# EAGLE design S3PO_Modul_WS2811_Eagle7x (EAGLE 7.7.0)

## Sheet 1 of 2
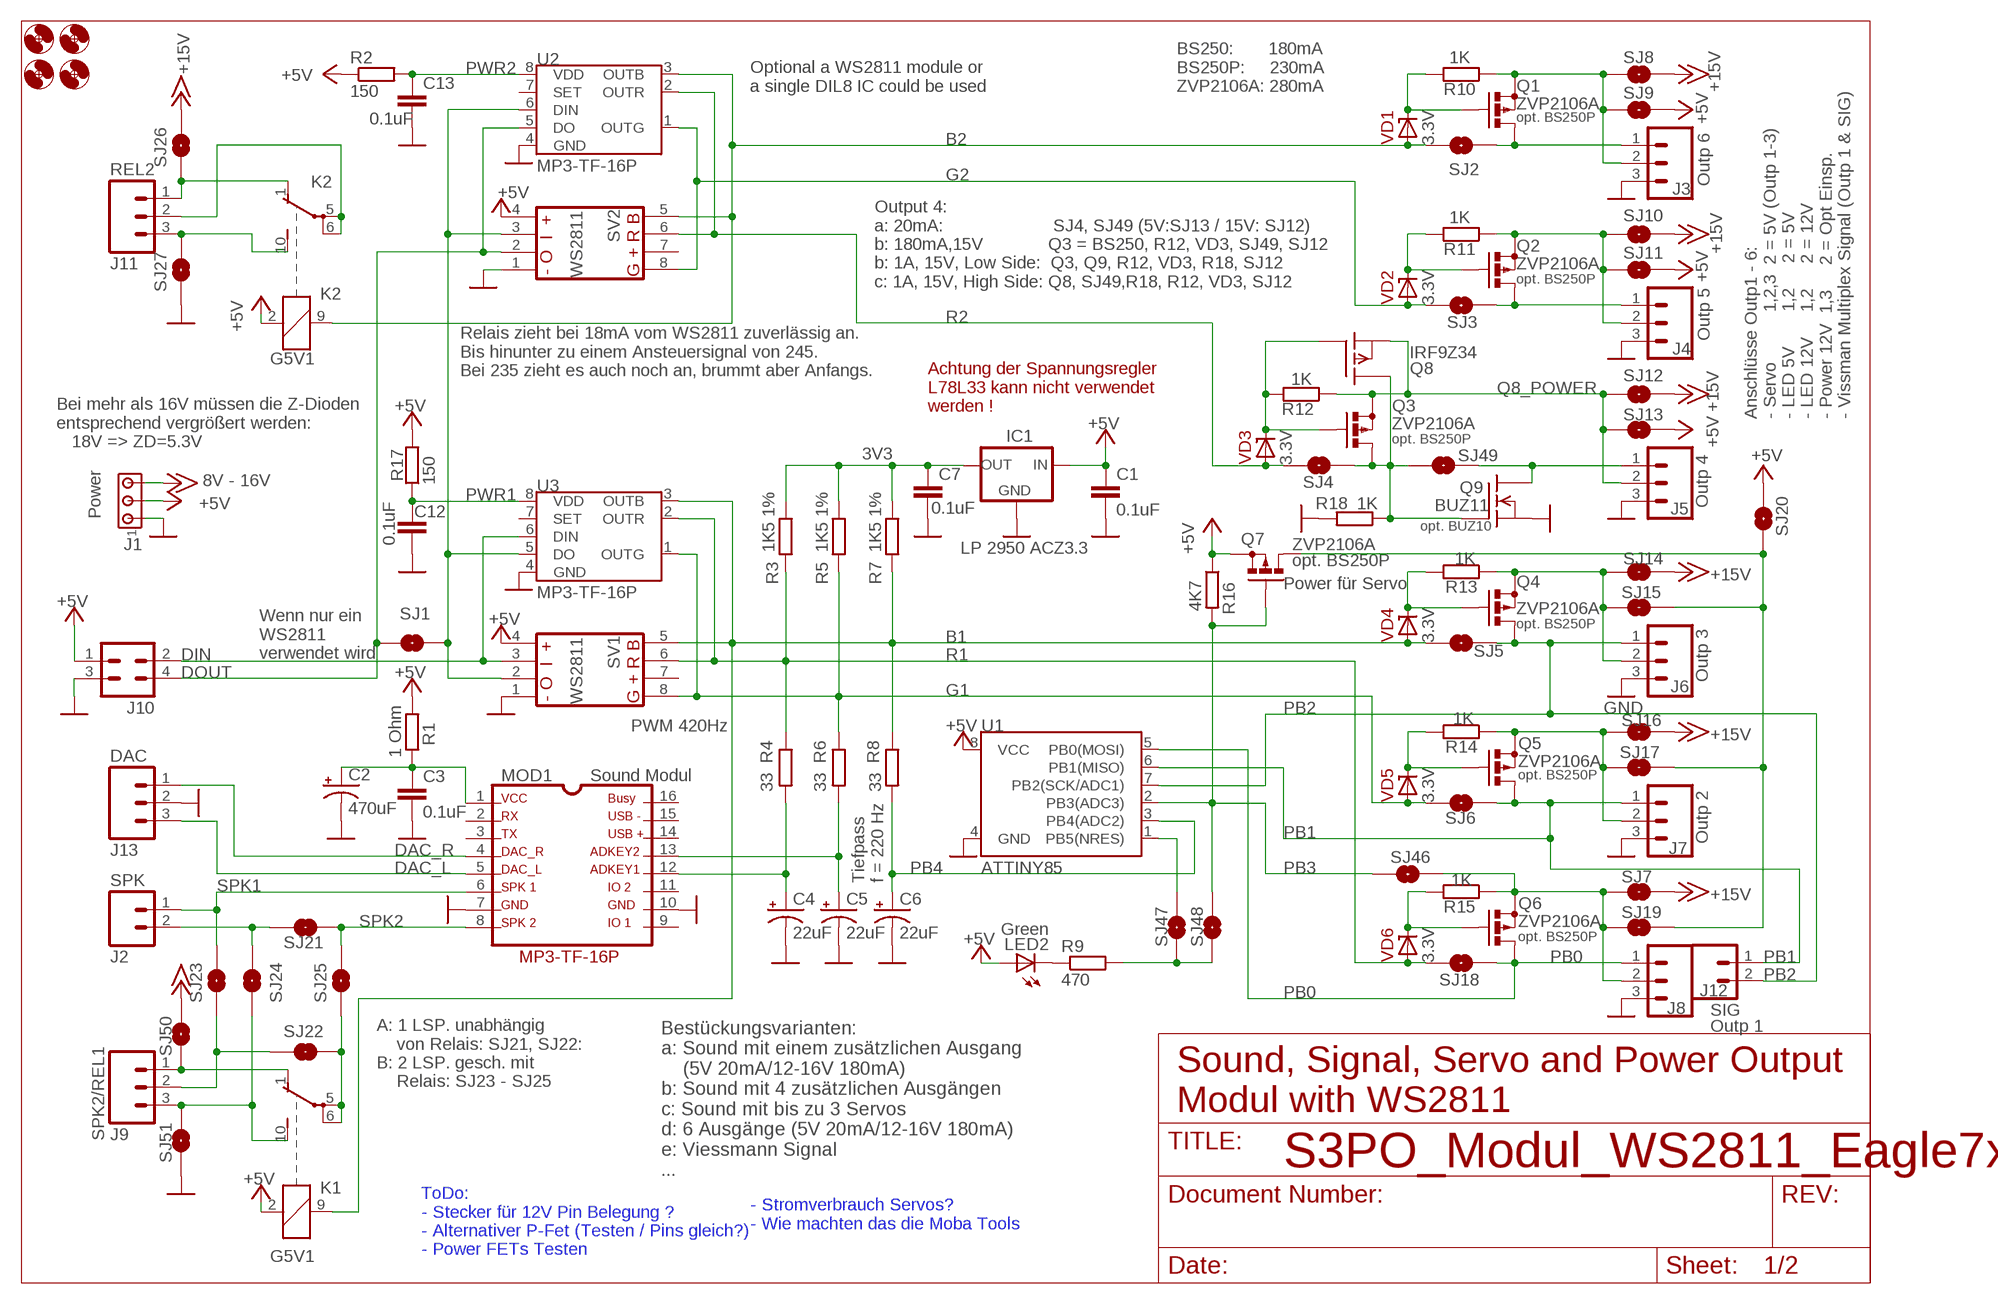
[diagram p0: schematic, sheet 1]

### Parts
C1  0.1uF  0.1UF-50V-20%(PTH)KIT-EZ  [CAP-PTH-SMALL-KIT]
C2  470uF  SPARKFUN-CAPACITORS_100UF-25V-20%(PTH)  [SPARKFUN-CAPACITORS_CPOL-RADIAL-100UF-25V]
C3  0.1uF  0.1UF-50V-20%(PTH)KIT-EZ  [CAP-PTH-SMALL-KIT]
C4  22uF  CAPACITORS_22UF  [CAPACITOR_CPOL-RADIAL-22UF]
C5  22uF  CAPACITORS_22UF  [CAPACITOR_CPOL-RADIAL-22UF]
C6  22uF  CAPACITORS_22UF  [CAPACITOR_CPOL-RADIAL-22UF]
C7  0.1uF  0.1UF-50V-20%(PTH)KIT-EZ  [CAP-PTH-SMALL-KIT]
C12  0.1uF  0.1UF-50V-20%(PTH)KIT-EZ  [CAP-PTH-SMALL-KIT]
C13  0.1uF  0.1UF-50V-20%(PTH)KIT-EZ  [CAP-PTH-SMALL-KIT]
H1  MOUNT-HOLE3.0  [3,0]
H2  MOUNT-HOLE3.0  [3,0]
H3  MOUNT-HOLE3.0  [3,0]
H4  MOUNT-HOLE3.0  [3,0]
IC1  LP 2950 ACZ3.3  78LXX  [78LXX]
J1  Power  MTA03-100  [10X03MTA]
J2  SPK  M02PTH  [1X02]
J3  Outp 6  M03PTH  [1X03]
J4  Outp 5  M03PTH  [1X03]
J5  Outp 4  M03PTH  [1X03]
J6  Outp 3  M03PTH  [1X03]
J7  Outp 2  M03PTH  [1X03]
J8  Outp 1  M03PTH  [1X03]
J9  SPK2/REL1  M03PTH  [1X03]
J10  INP  CON-HARTING-ML_ML4  [CON-HARTING-ML_ML4]
J11  REL2  M03PTH  [1X03]
J12  SIG  M02PTH  [1X02]
J13  DAC  M03PTH  [1X03]
K1  G5V1  [G5V1]
K2  G5V1  [G5V1]
LED2  Green  LED_LED3MM  [LED_LED3MM]
MOD1  Sound Modul  MP3-TF-16P_MP3-TF-16P  [MP3-TF-16P_MP3-TF-16P]
Q1  ZVP2106A  BS250  [SOT54E]
Q2  ZVP2106A  BS250  [SOT54E]
Q3  ZVP2106A  BS250  [SOT54E]
Q4  ZVP2106A  BS250  [SOT54E]
Q5  ZVP2106A  BS250  [SOT54E]
Q6  ZVP2106A  BS250  [SOT54E]
Q7  ZVP2106A  BS250  [SOT54E]
Q8  IRF9Z34  P-FET_IRF9Z34V  [TO220V]
Q9  BUZ11  N-FET_BUZ11V  [TO220V]
R1  1 Ohm  RCL_R-EU_0207/2V  [RCL_0207/2V]
R2  150  RCL_R-EU_0207/2V  [RCL_0207/2V]
R3  1K5 1%  RCL_R-EU_0204/5  [RCL_0204/5]
R4  33  RCL_R-EU_0204/5  [RCL_0204/5]
R5  1K5 1%  RCL_R-EU_0204/5  [RCL_0204/5]
R6  33  RCL_R-EU_0204/5  [RCL_0204/5]
R7  1K5 1%  RCL_R-EU_0204/5  [RCL_0204/5]
R8  33  RCL_R-EU_0204/5  [RCL_0204/5]
R9  470  RCL_R-EU_0207/2V  [RCL_0207/2V]
R10  1K  RCL_R-EU_0207/2V  [RCL_0207/2V]
R11  1K  RCL_R-EU_0207/2V  [RCL_0207/2V]
R12  1K  RCL_R-EU_0207/2V  [RCL_0207/2V]
R13  1K  RCL_R-EU_0207/2V  [RCL_0207/2V]
R14  1K  RCL_R-EU_0207/2V  [RCL_0207/2V]
R15  1K  RCL_R-EU_0207/2V  [RCL_0207/2V]
R16  4K7  RCL_R-EU_0207/2V  [RCL_0207/2V]
R17  150  RCL_R-EU_0207/2V  [RCL_0207/2V]
R18  1K  RCL_R-EU_0204/7  [RCL_0204/7]
SJ1  SOLDERJUMPERNO  [SJ_2S-NO]
SJ2  SOLDERJUMPERNO  [SJ_2S-NO]
SJ3  SOLDERJUMPERNO  [SJ_2S-NO]
SJ4  SOLDERJUMPERNO  [SJ_2S-NO]
SJ5  SOLDERJUMPERNO  [SJ_2S-NO]
SJ6  SOLDERJUMPERNO  [SJ_2S-NO]
SJ7  SOLDERJUMPERNO  [SJ_2S-NO]
SJ8  SOLDERJUMPERNO  [SJ_2S-NO]
SJ9  SOLDERJUMPERNO  [SJ_2S-NO]
SJ10  SOLDERJUMPERNO  [SJ_2S-NO]
SJ11  SOLDERJUMPERNO  [SJ_2S-NO]
SJ12  SOLDERJUMPERNO  [SJ_2S-NO]
SJ13  SOLDERJUMPERNO  [SJ_2S-NO]
SJ14  SOLDERJUMPERNO  [SJ_2S-NO]
SJ15  SOLDERJUMPERNO  [SJ_2S-NO]
SJ16  SOLDERJUMPERNO  [SJ_2S-NO]
SJ17  SOLDERJUMPERNO  [SJ_2S-NO]
SJ18  SOLDERJUMPERNO  [SJ_2S-NO]
SJ19  SOLDERJUMPERNO  [SJ_2S-NO]
SJ20  Servo Const 5V  SOLDERJUMPERNO  [SJ_2S-NO]
SJ21  SOLDERJUMPERNO  [SJ_2S-NO]
SJ22  SOLDERJUMPERNO  [SJ_2S-NO]
SJ23  SOLDERJUMPERNO  [SJ_2S-NO]
SJ24  SOLDERJUMPERNO  [SJ_2S-NO]
SJ25  SOLDERJUMPERNO  [SJ_2S-NO]
SJ26  SOLDERJUMPERNO  [SJ_2S-NO]
SJ27  SOLDERJUMPERNO  [SJ_2S-NO]
SJ46  Servo Const 5V  SOLDERJUMPERNO  [SJ_2S-NO]
SJ47  SOLDERJUMPERNO  [SJ_2S-NO]
SJ48  SOLDERJUMPERNO  [SJ_2S-NO]
SJ49  SOLDERJUMPERNO  [SJ_2S-NO]
SJ50  SOLDERJUMPERNO  [SJ_2S-NO]
SJ51  SOLDERJUMPERNO  [SJ_2S-NO]
SV1  S3PO_MODUL_WS2811_SOUND_MP3-TF-16P_WS2811_AND_ATTINY_PUSHBUTTONACTION_4017_2_WS28115V  [S3PO_MODUL_WS2811_SOUND_MP3-TF-16P_WS2811_AND_ATTINY_PUSHBUTTONACTION_4017_2_WS2811_WS2811_5V]
SV2  S3PO_MODUL_WS2811_SOUND_MP3-TF-16P_WS2811_AND_ATTINY_PUSHBUTTONACTION_4017_2_WS28115V  [S3PO_MODUL_WS2811_SOUND_MP3-TF-16P_WS2811_AND_ATTINY_PUSHBUTTONACTION_4017_2_WS2811_WS2811_5V]
U1  ATTINY85  ATTINY45TINY85-20-DIP  [DIP08]
U2  MP3-TF-16P  S3PO_MODUL_WS2811_SOUND_MP3-TF-16P_WS2811_AND_ATTINY_WS2811-ICTINY45-20-DIP  [S3PO_MODUL_WS2811_SOUND_MP3-TF-16P_WS2811_AND_ATTINY_WS2811_DIP08]
U3  MP3-TF-16P  S3PO_MODUL_WS2811_SOUND_MP3-TF-16P_WS2811_AND_ATTINY_WS2811-ICTINY45-20-DIP  [S3PO_MODUL_WS2811_SOUND_MP3-TF-16P_WS2811_AND_ATTINY_WS2811_DIP08]
VD1  3.3V  DIODES-ZENER_10V(1N4740)  [DIODES-ZENER_207/2V]
VD2  3.3V  DIODES-ZENER_10V(1N4740)  [DIODES-ZENER_207/2V]
VD3  3.3V  DIODES-ZENER_10V(1N4740)  [DIODES-ZENER_207/2V]
VD4  3.3V  DIODES-ZENER_10V(1N4740)  [DIODES-ZENER_207/2V]
VD5  3.3V  DIODES-ZENER_10V(1N4740)  [DIODES-ZENER_207/2V]
VD6  3.3V  DIODES-ZENER_10V(1N4740)  [DIODES-ZENER_207/2V]

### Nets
3V3: C7.1 IC1.OUT R3.1 R5.1 R7.1
+5V: C1.1 IC1.IN J1.2 J10.1 K1.2 K2.2 LED2.A Q7.S R1.1 R2.1 R16.1 R17.2 SJ9.2 SJ11.2 SJ13.2 SJ20.2 SV1.4(GND) SV2.4(GND) U1.8(VCC)
+15V: J1.3 SJ7.2 SJ8.2 SJ10.2 SJ12.2 SJ14.2 SJ16.2 SJ26.1 SJ50.1
B1: K1.9 R7.2 R8.1 SJ5.2 SV1.5(OUTG) U3.3(OUTB) VD4.A
B2: K2.9 SJ2.2 SV2.5(OUTG) U2.3(OUTB) VD1.A
DAC_L: J13.3 MOD1.5
DAC_R: J13.1 MOD1.4
DIN: J10.2 SV1.3(DO) U3.6(DIN)
DOUT: J10.4 SJ1.2 SV2.2(DIN) U2.5(DO)
G1: R5.2 R6.1 SJ6.2 SV1.8(OUTB) U3.1(OUTG) VD5.A
G2: SJ3.2 SV2.8(OUTB) U2.1(OUTG) VD2.A
GND: C1.2 C2.2(-) C3.2 C4.2(-) C5.2(-) C6.2(-) C7.2 C12.2 C13.2 IC1.GND J1.1 J3.3 J4.3 J5.3 J6.3 J7.3 J8.3 J10.3 J13.2 MOD1.7 MOD1.10 Q9.3(S) R18.2 SJ27.2 SJ51.2 SV1.1(VDD) SV2.1(VDD) U1.4(GND) U2.4(GND) U3.4(GND)
N$4: SJ1.1 SV1.2(DIN) SV2.3(DO) U2.6(DIN) U3.5(DO)
N$6: LED2.K(C) R9.1
N$7: C4.1(+) MOD1.12 R4.2
N$8: C5.1(+) MOD1.13 R6.2
N$9: C2.1(+) C3.1 MOD1.1 R1.2
N$10: Q4.G R13.2 VD4.C
N$14: J5.1 Q9.2(D) SJ49.2
N$17: Q6.G R15.2 VD6.C
N$18: Q3.D Q8.2(D) Q9.1(G) R18.1 SJ4.1 SJ49.1
N$19: Q3.G Q8.1(G) R12.2 VD3.C
N$21: J2.2 SJ21.2 SJ24.1
N$22: J4.1 Q2.D SJ3.1
N$23: Q2.G R11.2 VD2.C
N$24: J7.2 Q5.S R14.1 SJ16.1 SJ17.1
N$25: J8.2 Q6.S R15.1 SJ7.1 SJ19.1 SJ46.2
N$26: J3.1 Q1.D SJ2.1
N$27: Q1.G R10.2 VD1.C
N$29: K1.5(2:P) K1.6(2:P) SJ22.1 SJ25.2
N$32: Q5.G R14.2 VD5.C
N$34: J9.3 K1.10(2:S) SJ24.2 SJ51.1
N$35: J9.1 K1.1(2:O) SJ50.2
N$36: J9.2 SJ22.2 SJ23.2
N$37: J6.2 Q4.S R13.1 SJ14.1 SJ15.1
N$41: J4.2 Q2.S R11.1 SJ10.1 SJ11.1
N$42: J3.2 Q1.S R10.1 SJ8.1 SJ9.1
N$43: J11.2 K2.5(2:P) K2.6(2:P)
N$44: Q7.D SJ15.2 SJ17.2 SJ19.2 SJ20.1
N$45: J11.3 K2.10(2:S) SJ27.1
N$46: J11.1 K2.1(2:O) SJ26.2
N$70: SJ47.2 U1.1(PB5(NRES))
N$74: R9.2 SJ47.1 SJ48.2
PB0: J8.1 Q6.D SJ18.1 U1.5(PB0(MOSI))
PB1: J7.1 J12.1 Q5.D SJ6.1 U1.6(PB1(MISO))
PB2: J6.1 J12.2 Q4.D SJ5.1 U1.7(PB2(SCK/ADC1))
PB3: Q7.G R16.2 SJ46.1 SJ48.1 U1.2(PB3(ADC3))
PB4: C6.1(+) R8.2 U1.3(PB4(ADC2))
PWR1: C12.1 R17.1 U3.8(VDD)
PWR2: C13.1 R2.2 U2.8(VDD)
Q8_POWER: J5.2 Q3.S Q8.3(S) R12.1 SJ12.1 SJ13.1
R1: R3.2 R4.1 SJ18.2 SV1.6(OUT+) U3.2(OUTR) VD6.A
R2: SJ4.2 SV2.6(OUT+) U2.2(OUTR) VD3.A
SPK1: J2.1 MOD1.6 SJ23.1
SPK2: MOD1.8 SJ21.1 SJ25.1
Unconnected: MOD1.2 MOD1.3 MOD1.9 MOD1.11 MOD1.14 MOD1.15 MOD1.16 SV1.7(OUTR) SV2.7(OUTR) U2.7(SET) U3.7(SET)

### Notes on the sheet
- Optional a WS2811 module or
  a single DIL8 IC could be used
- BS250:       180mA
  BS250P:     230mA
  ZVP2106A: 280mA
- opt. BS250P
- opt. BS250P
- Output 4:
  a: 20mA:                      SJ4, SJ49 (5V:SJ13 / 15V: SJ12) 
  b: 180mA,15V             Q3 = BS250, R12, VD3, SJ49, SJ12
  b: 1A, 15V, Low Side:  Q3, Q9, R12, VD3, R18, SJ12
  c: 1A, 15V, High Side: Q8, SJ49,R18, R12, VD3, SJ12
- Relais zieht bei 18mA vom WS2811 zuverlässig an.
  Bis hinunter zu einem Ansteuersignal von 245.
  Bei 235 zieht es auch noch an, brummt aber Anfangs.
- Achtung der Spannungsregler
  L78L33 kann nicht verwendet
  werden !
- Anschlüsse Outp1 - 6:
  - Servo          1,2,3  2 = 5V (Outp 1-3)
  - LED 5V       1,2     2 = 5V
  - LED 12V     1,2     2 = 12V
  - Power 12V  1,3     2 = Opt Einsp.
  - Vissman Multiplex Signal (Outp 1 & SIG)
- opt. BS250P
- Bei mehr als 16V müssen die Z-Dioden
  entsprechend vergrößert werden: 
     18V => ZD=5.3V
- 8V - 16V
- opt. BUZ10
- opt. BS250P
- Power für Servo
- opt. BS250P
- Wenn nur ein  
  WS2811 
  verwendet wird
- PWM 420Hz
- opt. BS250P
- Tiefpass 
  f = 220 Hz
- opt. BS250P
- A: 1 LSP. unabhängig
      von Relais: SJ21, SJ22: 
  B: 2 LSP. gesch. mit
      Relais: SJ23 - SJ25
- Sound, Signal, Servo and Power Output
  Modul with WS2811
- Bestückungsvarianten:
  a: Sound mit einem zusätzlichen Ausgang 
      (5V 20mA/12-16V 180mA)
  b: Sound mit 4 zusätzlichen Ausgängen          
  c: Sound mit bis zu 3 Servos 
  d: 6 Ausgänge (5V 20mA/12-16V 180mA)
  e: Viessmann Signal
  ...
- - Stromverbrauch Servos? 
  - Wie machten das die Moba Tools
- ToDo:
  - Stecker für 12V Pin Belegung ?
  - Alternativer P-Fet (Testen / Pins gleich?)
  - Power FETs Testen

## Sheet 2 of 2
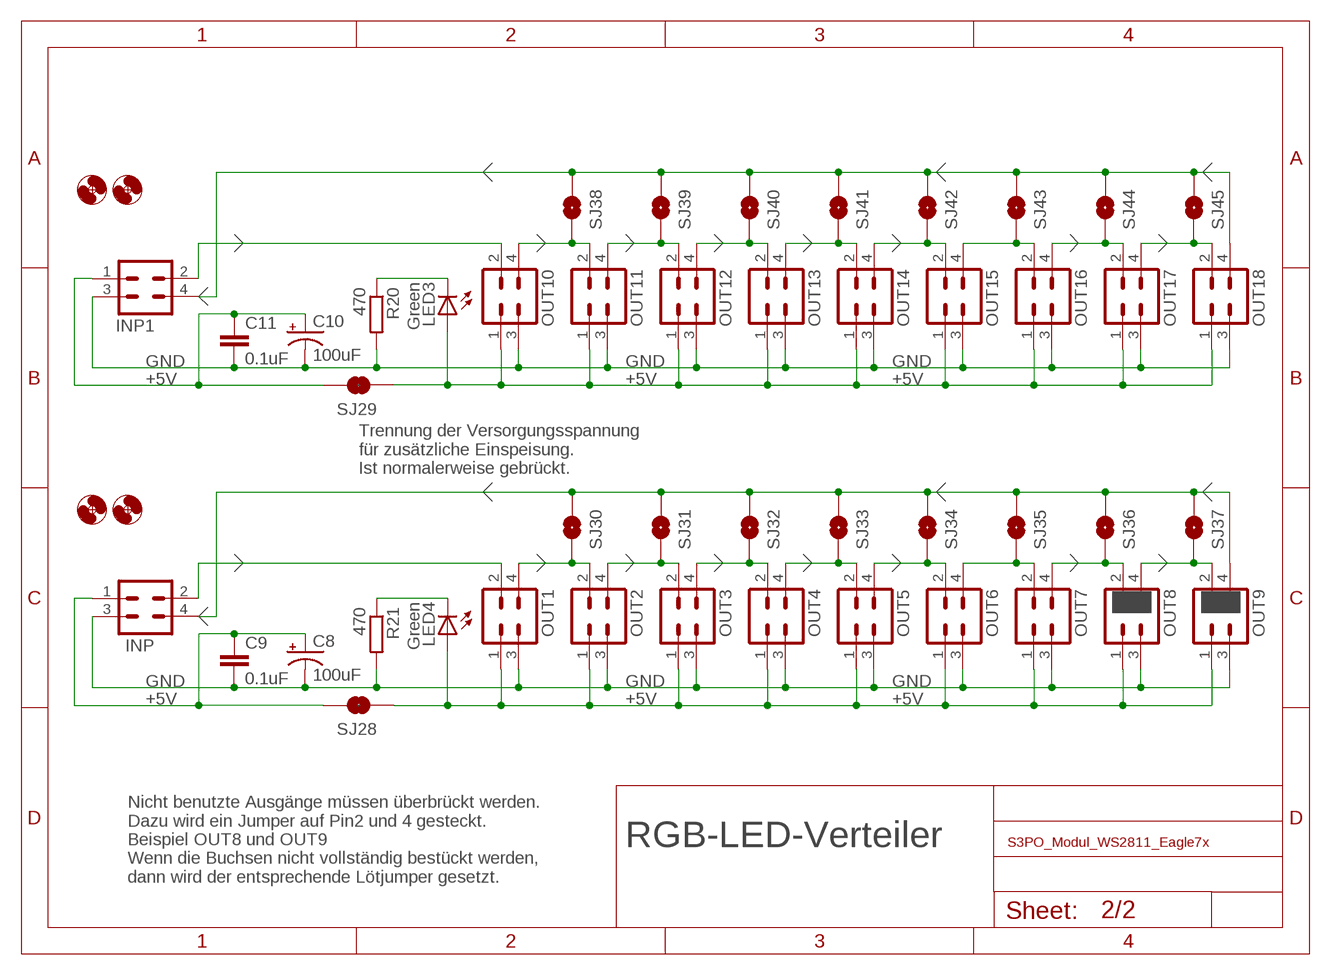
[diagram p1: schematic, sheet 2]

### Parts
C8  100uF  SPARKFUN-CAPACITORS_100UF-25V-20%(PTH)  [SPARKFUN-CAPACITORS_CPOL-RADIAL-100UF-25V]
C9  0.1uF  0.1UF-50V-20%(PTH)KIT-EZ  [CAP-PTH-SMALL-KIT]
C10  100uF  SPARKFUN-CAPACITORS_100UF-25V-20%(PTH)  [SPARKFUN-CAPACITORS_CPOL-RADIAL-100UF-25V]
C11  0.1uF  0.1UF-50V-20%(PTH)KIT-EZ  [CAP-PTH-SMALL-KIT]
H5  MOUNT-HOLE3.0  [3,0]
H6  MOUNT-HOLE3.0  [3,0]
H7  MOUNT-HOLE3.0  [3,0]
H8  MOUNT-HOLE3.0  [3,0]
INP  CON-HARTING-ML_ML4  [CON-HARTING-ML_ML4]
INP1  CON-HARTING-ML_ML4  [CON-HARTING-ML_ML4]
LED3  Green  LED_LED3MM  [LED_LED3MM]
LED4  Green  LED_LED3MM  [LED_LED3MM]
OUT1  CON-HARTING-ML_ML4  [CON-HARTING-ML_ML4]
OUT2  CON-HARTING-ML_ML4  [CON-HARTING-ML_ML4]
OUT3  CON-HARTING-ML_ML4  [CON-HARTING-ML_ML4]
OUT4  CON-HARTING-ML_ML4  [CON-HARTING-ML_ML4]
OUT5  CON-HARTING-ML_ML4  [CON-HARTING-ML_ML4]
OUT6  CON-HARTING-ML_ML4  [CON-HARTING-ML_ML4]
OUT7  CON-HARTING-ML_ML4  [CON-HARTING-ML_ML4]
OUT8  CON-HARTING-ML_ML4  [CON-HARTING-ML_ML4]
OUT9  CON-HARTING-ML_ML4  [CON-HARTING-ML_ML4]
OUT10  CON-HARTING-ML_ML4  [CON-HARTING-ML_ML4]
OUT11  CON-HARTING-ML_ML4  [CON-HARTING-ML_ML4]
OUT12  CON-HARTING-ML_ML4  [CON-HARTING-ML_ML4]
OUT13  CON-HARTING-ML_ML4  [CON-HARTING-ML_ML4]
OUT14  CON-HARTING-ML_ML4  [CON-HARTING-ML_ML4]
OUT15  CON-HARTING-ML_ML4  [CON-HARTING-ML_ML4]
OUT16  CON-HARTING-ML_ML4  [CON-HARTING-ML_ML4]
OUT17  CON-HARTING-ML_ML4  [CON-HARTING-ML_ML4]
OUT18  CON-HARTING-ML_ML4  [CON-HARTING-ML_ML4]
R20  470  RCL_R-EU_0207/2V  [RCL_0207/2V]
R21  470  RCL_R-EU_0207/2V  [RCL_0207/2V]
SJ28  SOLDERJUMPERTRACE  [SJ_2S-TRACE]
SJ29  SOLDERJUMPERTRACE  [SJ_2S-TRACE]
SJ30  SOLDERJUMPERNO  [SJ_2S-NO]
SJ31  SOLDERJUMPERNO  [SJ_2S-NO]
SJ32  SOLDERJUMPERNO  [SJ_2S-NO]
SJ33  SOLDERJUMPERNO  [SJ_2S-NO]
SJ34  SOLDERJUMPERNO  [SJ_2S-NO]
SJ35  SOLDERJUMPERNO  [SJ_2S-NO]
SJ36  SOLDERJUMPERNO  [SJ_2S-NO]
SJ37  SOLDERJUMPERNO  [SJ_2S-NO]
SJ38  SOLDERJUMPERNO  [SJ_2S-NO]
SJ39  SOLDERJUMPERNO  [SJ_2S-NO]
SJ40  SOLDERJUMPERNO  [SJ_2S-NO]
SJ41  SOLDERJUMPERNO  [SJ_2S-NO]
SJ42  SOLDERJUMPERNO  [SJ_2S-NO]
SJ43  SOLDERJUMPERNO  [SJ_2S-NO]
SJ44  SOLDERJUMPERNO  [SJ_2S-NO]
SJ45  SOLDERJUMPERNO  [SJ_2S-NO]

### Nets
5V_A: LED4.A OUT1.1 OUT2.1 OUT3.1 OUT4.1 OUT5.1 OUT6.1 OUT7.1 OUT8.1 OUT9.1 SJ28.1
5V_B: LED3.A OUT10.1 OUT11.1 OUT12.1 OUT13.1 OUT14.1 OUT15.1 OUT16.1 OUT17.1 OUT18.1 SJ29.1
GND_A: C8.2(-) C9.2 INP.3 OUT1.3 OUT2.3 OUT3.3 OUT4.3 OUT5.3 OUT6.3 OUT7.3 OUT8.3 OUT9.3 R21.2
GND_B: C10.2(-) C11.2 INP1.3 OUT10.3 OUT11.3 OUT12.3 OUT13.3 OUT14.3 OUT15.3 OUT16.3 OUT17.3 OUT18.3 R20.2
N$5: LED3.K(C) R20.1
N$11: OUT1.4 OUT2.2 SJ30.2
N$12: OUT2.4 OUT3.2 SJ31.2
N$16: LED4.K(C) R21.1
N$47: OUT3.4 OUT4.2 SJ32.2
N$48: INP.2 OUT1.2
N$49: OUT10.4 OUT11.2 SJ38.2
N$50: OUT4.4 OUT5.2 SJ33.2
N$51: OUT5.4 OUT6.2 SJ34.2
N$54: OUT11.4 OUT12.2 SJ39.2
N$55: OUT7.4 OUT8.2 SJ36.2
N$56: INP.4 OUT9.4 SJ30.1 SJ31.1 SJ32.1 SJ33.1 SJ34.1 SJ35.1 SJ36.1 SJ37.1
N$57: OUT8.4 OUT9.2 SJ37.2
N$58: OUT12.4 OUT13.2 SJ40.2
N$59: INP1.2 OUT10.2
N$60: OUT13.4 OUT14.2 SJ41.2
N$61: OUT6.4 OUT7.2 SJ35.2
N$62: OUT14.4 OUT15.2 SJ42.2
N$65: OUT16.4 OUT17.2 SJ44.2
N$66: INP1.4 OUT18.4 SJ38.1 SJ39.1 SJ40.1 SJ41.1 SJ42.1 SJ43.1 SJ44.1 SJ45.1
N$67: OUT17.4 OUT18.2 SJ45.2
N$68: OUT15.4 OUT16.2 SJ43.2
N$69: C8.1(+) C9.1 INP.1 SJ28.2
N$73: C10.1(+) C11.1 INP1.1 SJ29.2

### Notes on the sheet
- GND | GND | GND
- +5V | +5V | +5V
- Trennung der Versorgungsspannung
  für zusätzliche Einspeisung.
  Ist normalerweise gebrückt.
- GND | GND | GND
- +5V | +5V | +5V
- RGB-LED-Verteiler
- Nicht benutzte Ausgänge müssen überbrückt werden.
  Dazu wird ein Jumper auf Pin2 und 4 gesteckt.
  Beispiel OUT8 und OUT9
  Wenn die Buchsen nicht vollständig bestückt werden, 
  dann wird der entsprechende Lötjumper gesetzt.

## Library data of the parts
C1 C3 C7 C9 C11-C13 = SparkFun-Capacitors:0.1UF-50V-20%(PTH): CAP-08370; PROD_ID: CAP-08370
C2 C8 C10 = Sound_MP3-TF-16P_and_WS2811:SPARKFUN-CAPACITORS_100UF-25V-20%(PTH): CAP-08439; PROD_ID: CAP-08439
C4-C6 = Sound_MP3-TF-16P_WS2811_and_ATTiny:CAPACITORS_22UF: CAP-08439; PROD_ID: CAP-08439
H1-H8 = holes:MOUNT-HOLE: MOUNTING HOLE with drill center marker
IC1 = v-reg-3:78LXX: VOLTAGE REGULATOR
INP INP1 OUT1-OUT18 = RGB-LED-Verteiler:CON-HARTING-ML_ML4
J1 = con-amp:MTA03-100: AMP connector
J2 J12 = SparkFun-Connectors:M02: Standard 2-pin 0.1" header. Use with
J3-J9 J11 J13 = SparkFun-Connectors:M03: Header 3 Standard 3-pin 0.1" header. Use with straight break away headers (SKU : PRT-00116), right angle break away headers (PRT-00553), swiss pins (PRT-00743), machine pins (PRT-00117), and female headers (PRT-00115). Molex polarized connector foot print use with SKU : PRT-08232 with associated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
J10 = Pfostenstecker_4_u_6:CON-HARTING-ML_ML4
K1 K2 = relay:G5V1: RELAY 1 x switch, 0.5 A/125 V AC, 1 A/24 V DC , Omron; MPN: G5V-1-DC24; OC_FARNELL: 9949593; OC_NEWARK: 36M6377; SPICEPREFIX: B
LED2-LED4 = Sound_MP3-TF-16P_and_WS2811:LED_LED: LED
MOD1 = Sound_MP3-TF-16P_WS2811_and_ATTiny:MP3-TF-16P_MP3-TF-16P: MP3-TF-16P http://www.electronicoscaldas.com/datasheet/DFR0299-DFPlayer-Mini-Manual.pdf; OC_FARNELL: unknown; OC_NEWARK: unknown
Q1-Q7 = transistor-small-signal:BS250: P-CHANNEL MOS FET
Q8 = S3PO_Modul_WS2811:P-FET_IRF9Z34
Q9 = S3PO_Modul_WS2811:N-FET_BUZ11: N-Channel Enhancement MOSFET 50V; 30A; 0,040Ohm
R1-R18 R20 R21 = Sound_MP3-TF-16P_and_WS2811:RCL_R-EU_: RESISTOR, European symbol; SPICEPREFIX: R
SJ1-SJ51 = SparkFun-Retired:SOLDERJUMPER: Solder Jumper
SV1 SV2 = S3PO_Modul_WS2811:S3PO_MODUL_WS2811_SOUND_MP3-TF-16P_WS2811_AND_ATTINY_PUSHBUTTONACTION_4017_2_WS2811: Modified by Hardi
U1 = SparkFun-DigitalIC:ATTINY45: Atmel 8-pin 2/4/8kB flash uC; PROD_ID: IC-09445; VALUE: TINY85-20-DIP
U2 U3 = S3PO_Modul_WS2811:S3PO_MODUL_WS2811_SOUND_MP3-TF-16P_WS2811_AND_ATTINY_WS2811-IC: Die Pin nummern im Dokument https://cdn-shop.adafruit.com/datasheets/WS2811.pdf für R und G sind vertauscht ;-(; PROD_ID: IC-09439; VALUE: TINY45-20-DIP
VD1-VD6 = Z-Diode:DIODES-ZENER_?

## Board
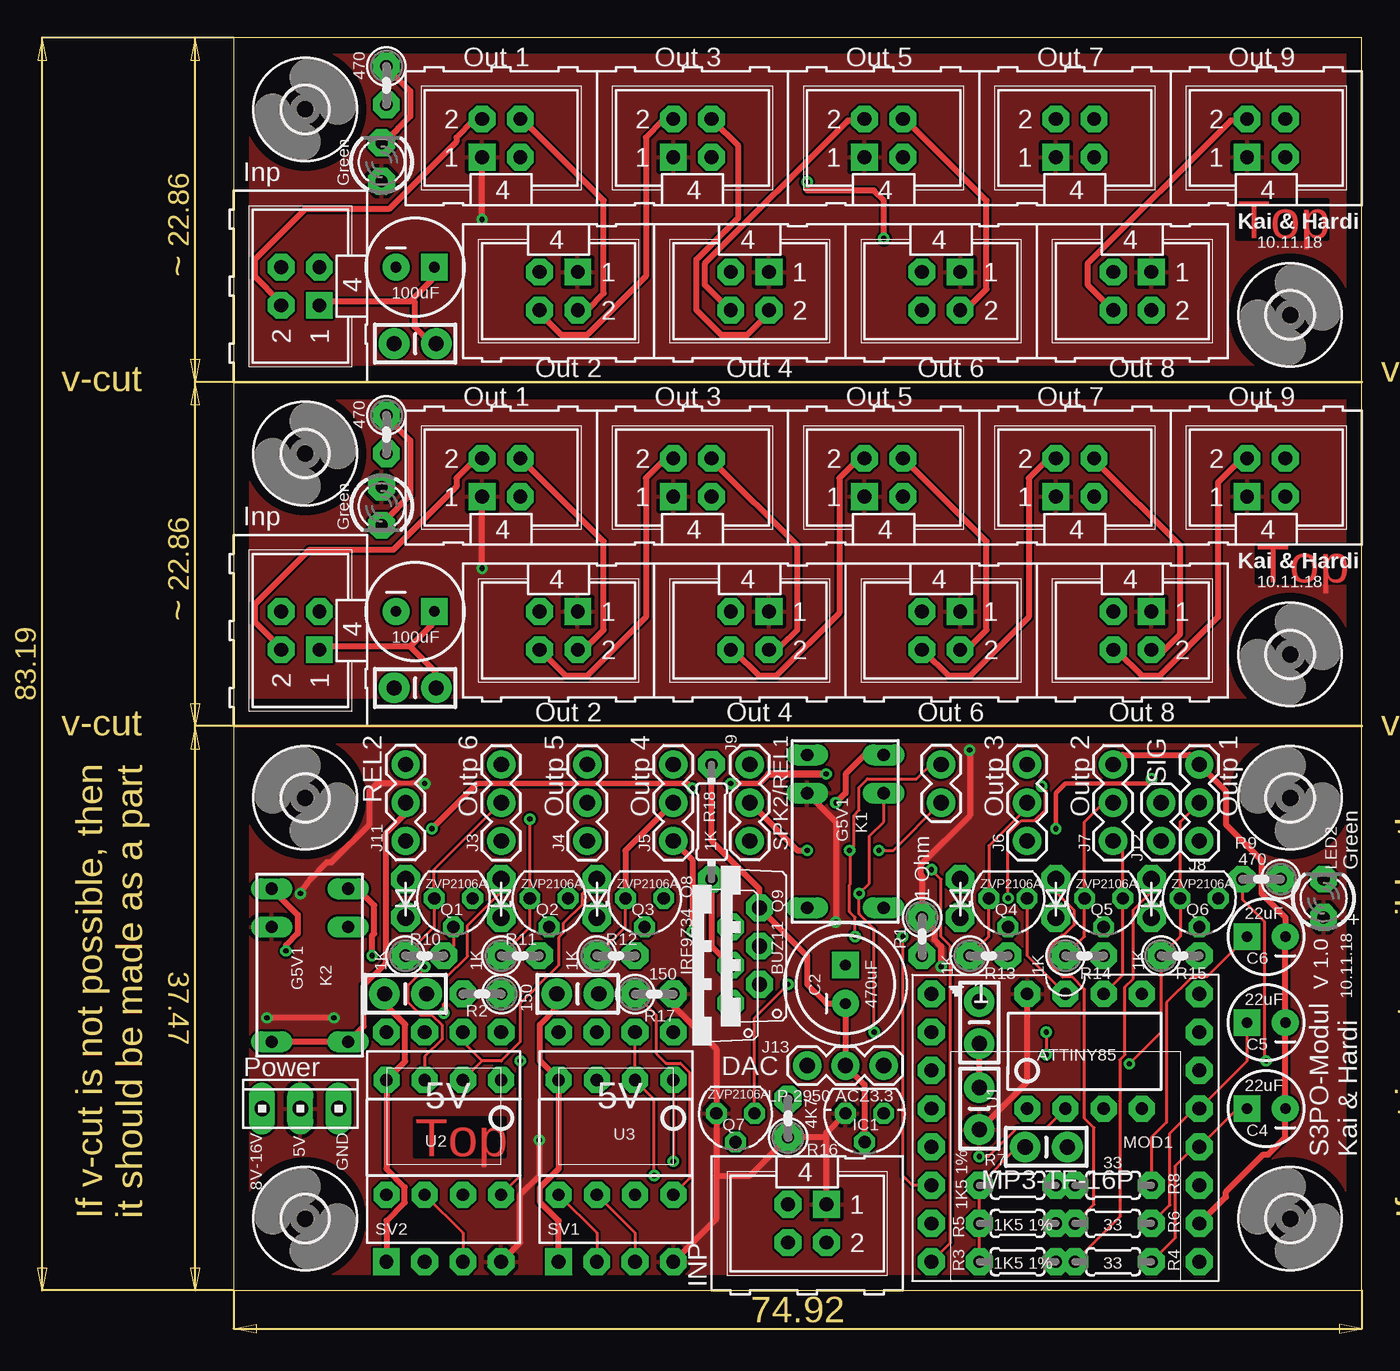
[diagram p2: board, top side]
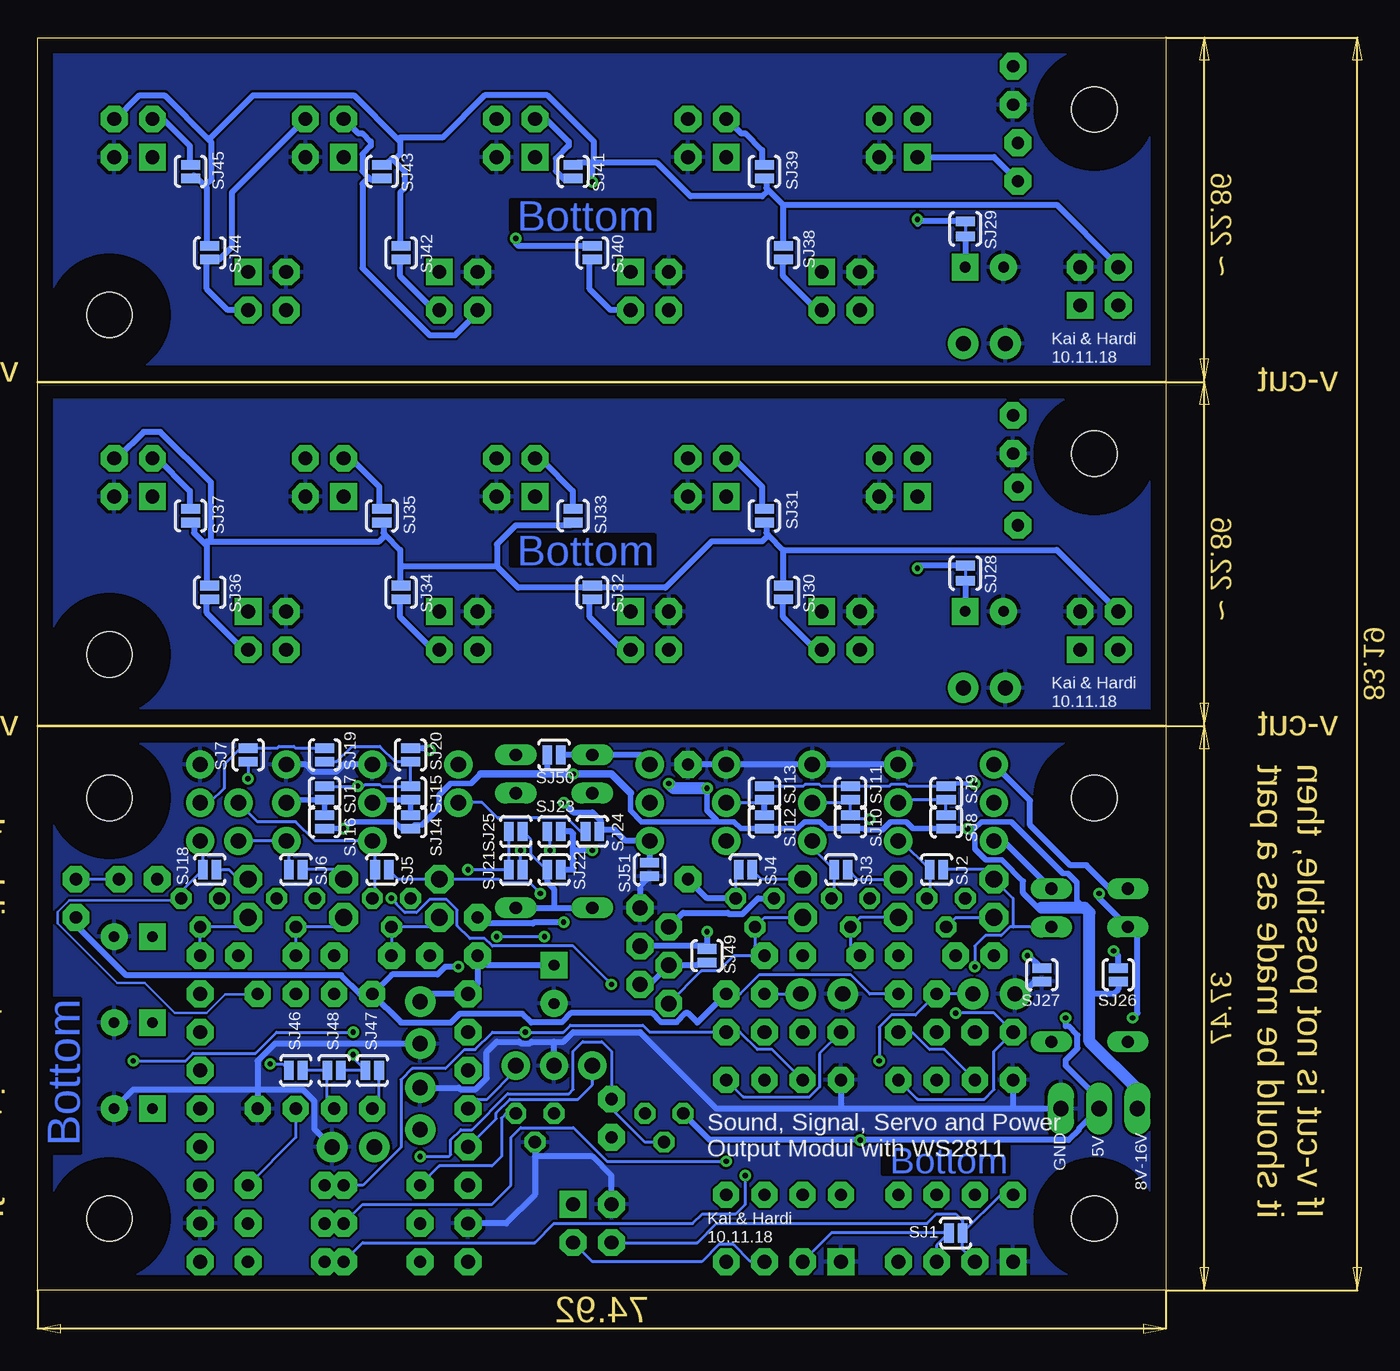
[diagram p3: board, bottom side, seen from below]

Size 87.93 x 86.03 mm. Coordinates in mm from the lower left corner, seen from the top.
Outline: 87.93,40.31 87.93,2.84 13.01,2.84 13.01,86.03 87.93,86.03 87.93,63.17
Outline: 87.93,40.31 87.93,63.17
Outline: 13,40.31 87.93,40.31
Outline: 13,63.17 87.93,63.17
Copper layers (1*16): Top 0.035mm / dielectric 1.5mm / Bottom 0.035mm
Design rules "default *": minimum track width 6mil, minimum drill 0.35mm, track to track 6mil, track to pad 6mil, pad to pad 6mil, via to via 6mil, smd to smd 6mil, copper to edge 40mil, drill to drill 6mil, minimum pad ring 10mil, minimum via ring 8mil, stop-mask expansion 4mil, vias tented up to drill 0mil, thermal gap 10mil

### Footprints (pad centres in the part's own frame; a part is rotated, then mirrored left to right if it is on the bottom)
CAP-PTH-SMALL-KIT = drill 1.016 pad 2.032: 1 -1.397,0; 2 1.397,0
SPARKFUN-CAPACITORS_CPOL-RADIAL-100UF-25V = drill 0.7 pad 1.778 square: 1 1.27,0 | drill 0.7 pad 1.778: 2 -1.27,0
CAPACITOR_CPOL-RADIAL-22UF = drill 0.7 pad 1.778 square: 1 1.27,0 | drill 0.7 pad 1.778: 2 -1.27,0
3,0 = hole 3: 0,0
78LXX = drill 0.813 octagon: GND 0,1.905; IN 1.27,0; OUT -1.27,0
CON-HARTING-ML_ML4 = drill 0.914 pad 1.778 square: 1 -2.54,-1.27 | drill 0.914 pad 1.778 octagon: 2 -2.54,1.27; 3 0,-1.27; 4 0,1.27
10X03MTA = drill 1.016 long: 1 2.54,0; 2 0,0; 3 -2.54,0
1X02 = drill 1.016 pad 1.88: 1 0,0; 2 2.54,0
1X03 = drill 1.016 pad 1.88: 1 0,0; 2 2.54,0; 3 5.08,0
G5V1 = drill 0.813 long: 1 -5.08,-2.54; 2 -2.54,-2.54; 5 5.08,-2.54; 6 5.08,2.54; 9 -2.54,2.54; 10 -5.08,2.54
LED_LED3MM = drill 0.813 pad 1.778 octagon: A -1.27,0; K 1.27,0
MP3-TF-16P_MP3-TF-16P = drill 0.914 pad 1.778 octagon: 1 -8.89,16.51; 2 -8.89,13.97; 3 -8.89,11.43; 4 -8.89,8.89; 5 -8.89,6.35; 6 -8.89,3.81; 7 -8.89,1.27; 8 -8.89,-1.27; 9 8.89,-1.27; 10 8.89,1.27; 11 8.89,3.81; 12 8.89,6.35; 13 8.89,8.89; 14 8.89,11.43; 15 8.89,13.97; 16 8.89,16.51
SOT54E = drill 0.813 octagon: D -1.27,0; G 0,1.905; S 1.27,0
TO220V = drill 1.016 pad 1.778 octagon: 1 -2.54,-2.54; 2 0,-2.54; 3 2.54,-2.54
RCL_0207/2V = drill 0.813 pad 1.778 octagon: 1 -1.27,0; 2 1.27,0
RCL_0204/5 = drill 0.813 pad 1.778 octagon: 1 -2.54,0; 2 2.54,0
RCL_0204/7 = drill 0.813 pad 1.778 octagon: 1 -3.81,0; 2 3.81,0
SJ_2S-NO = smd 0.635 x 1.27: 1 -0.45,0; 2 0.45,0
SJ_2S-TRACE = smd 0.635 x 1.27: 1 -0.508,0; 2 0.508,0
S3PO_MODUL_WS2811_SOUND_MP3-TF-16P_WS2811_AND_ATTINY_PUSHBUTTONACTION_4017_2_WS2811_WS2811_5V = drill 0.914 pad 1.778 square: 1 -5.08,-5.08 | drill 0.914 pad 1.778 octagon: 2 -2.54,-5.08; 3 0,-5.08; 4 2.54,-5.08; 5 2.54,10.16; 6 0,10.16; 7 -2.54,10.16; 8 -5.08,10.16
DIP08 = drill 0.813 pad 1.727 octagon: 1 -3.81,-3.81; 2 -1.27,-3.81; 3 1.27,-3.81; 4 3.81,-3.81; 5 3.81,3.81; 6 1.27,3.81; 7 -1.27,3.81; 8 -3.81,3.81
S3PO_MODUL_WS2811_SOUND_MP3-TF-16P_WS2811_AND_ATTINY_WS2811_DIP08 = drill 0.813 pad 1.727 octagon: 1 -3.81,-3.81; 2 -1.27,-3.81; 3 1.27,-3.81; 4 3.81,-3.81; 5 3.81,3.81; 6 1.27,3.81; 7 -1.27,3.81; 8 -3.81,3.81
DIODES-ZENER_207/2V = drill 1.118 pad 1.778 octagon: A 1.27,0; C -1.27,0

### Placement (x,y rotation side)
C1  62.53,14.9 90 top
C2  53.64,23.16 90 top
C3  62.53,20.62 270 top
C4  81.58,14.9 180 top
C5  81.58,20.62 180 top
C6  81.58,26.34 180 top
C7  66.97,12.37 0 top
C8  25.06,47.92 0 top
C9  25.06,42.84 180 top
C10  25.06,70.78 0 top
C11  25.06,65.7 180 top
C12  35.86,22.52 180 top
C13  24.43,22.52 180 top
H1  83.17,35.54 90 top
H2  83.17,7.6 90 top
H3  17.76,35.54 90 top
H4  17.76,7.6 90 top
H5  17.76,58.4 0 top
H6  83.17,45.07 0 top
H7  17.76,81.26 0 top
H8  83.17,67.61 0 top
IC1  54.91,14.59 180 top
INP  17.45,47.92 90 top
INP1  17.45,70.78 90 top
J1  17.45,14.9 0 top
J2  59.99,37.77 270 top
J3  30.78,32.69 90 top
J4  36.5,32.69 90 top
J5  42.21,32.69 90 top
J6  65.7,32.69 90 top
J7  71.42,32.69 90 top
J8  77.14,32.69 90 top
J9  47.29,37.77 270 top
J10  49.83,7.29 180 top
J11  24.43,37.77 270 top
J12  74.59,32.69 90 top
J13  56.18,17.76 180 top
K1  53.64,33.32 270 top
K2  18.08,24.43 270 top
LED2  85.39,28.88 90 top
LED3  22.84,77.77 90 top
LED4  22.84,54.91 270 top
MOD1  68.25,6.01 0 top
OUT1  32.05,56.81 0 top
OUT2  33.32,46.66 180 top
OUT3  44.75,56.81 0 top
OUT4  46.02,46.66 180 top
OUT5  57.45,56.81 0 top
OUT6  58.72,46.66 180 top
OUT7  70.15,56.81 0 top
OUT8  71.42,46.66 180 top
OUT9  82.85,56.81 0 top
OUT10  32.05,79.36 0 top
OUT11  33.32,69.2 180 top
OUT12  44.75,79.36 0 top
OUT13  46.02,69.2 180 top
OUT14  57.45,79.36 0 top
OUT15  58.72,69.2 180 top
OUT16  70.15,79.36 0 top
OUT17  71.42,69.2 180 top
OUT18  82.85,79.36 0 top
Q1  27.61,28.88 180 top
Q2  33.95,28.88 180 top
Q3  40.3,28.88 180 top
Q4  64.44,28.88 180 top
Q5  70.78,28.88 180 top
Q6  77.14,28.88 180 top
Q7  46.34,14.59 180 top
Q8  43.48,24.43 90 top
Q9  45.38,25.7 90 top
R1  58.72,26.34 270 top
R2  29.51,22.52 180 top
R3  65.07,4.75 0 top
R4  71.42,4.75 0 top
R5  65.07,7.29 0 top
R6  71.42,7.29 0 top
R7  65.07,9.82 0 top
R8  71.42,9.82 0 top
R9  81.26,30.14 180 top
R10  25.7,25.07 0 top
R11  32.05,25.07 0 top
R12  38.4,25.07 0 top
R13  63.16,25.07 0 top
R14  69.52,25.07 0 top
R15  75.87,25.07 0 top
R16  49.83,14.27 90 top
R17  40.94,22.52 0 top
R18  44.75,33.95 90 top
R20  23.16,82.85 270 top
R21  23.16,59.67 270 top
SJ1  26.97,6.65 0 bottom
SJ2  28.24,30.78 0 bottom
SJ3  34.59,30.78 0 bottom
SJ4  40.94,30.78 0 bottom
SJ5  65.07,30.78 0 bottom
SJ6  70.78,30.78 0 bottom
SJ7  73.96,38.4 270 bottom
SJ8  27.61,33.95 270 bottom
SJ9  27.61,35.86 90 bottom
SJ10  33.95,33.95 270 bottom
SJ11  33.95,35.86 90 bottom
SJ12  39.67,33.95 270 bottom
SJ13  39.67,35.86 90 bottom
SJ14  63.16,33.95 270 bottom
SJ15  63.16,35.86 90 bottom
SJ16  68.88,33.95 270 bottom
SJ17  68.88,35.86 90 bottom
SJ18  76.5,30.78 0 bottom
SJ19  68.88,38.4 270 bottom
SJ20  63.16,38.4 90 bottom
SJ21  56.18,30.78 0 bottom
SJ22  53.64,30.78 0 bottom
SJ23  53.64,33.32 0 bottom
SJ24  51.1,33.32 0 bottom
SJ25  56.18,33.32 0 bottom
SJ26  16.18,23.79 90 bottom
SJ27  21.26,23.79 270 bottom
SJ28  26.34,50.47 270 bottom
SJ29  26.34,73.33 270 bottom
SJ30  38.4,49.19 270 bottom
SJ31  39.67,54.28 90 bottom
SJ32  51.1,49.19 270 bottom
SJ33  52.37,54.28 90 bottom
SJ34  63.8,49.19 270 bottom
SJ35  65.07,54.28 90 bottom
SJ36  76.5,49.19 270 bottom
SJ37  77.77,54.28 90 bottom
SJ38  38.4,71.74 270 bottom
SJ39  39.67,77.14 90 bottom
SJ40  51.1,71.74 270 bottom
SJ41  52.37,77.14 270 bottom
SJ42  63.8,71.74 270 bottom
SJ43  65.07,77.14 270 bottom
SJ44  76.5,71.74 270 bottom
SJ45  77.77,77.14 90 bottom
SJ46  70.78,17.45 180 bottom
SJ47  65.7,17.45 0 bottom
SJ48  68.25,17.45 0 bottom
SJ49  43.48,25.07 90 bottom
SJ50  53.64,38.4 0 bottom
SJ51  47.29,30.78 270 bottom
SV1  39.67,9.82 0 top
SV2  28.24,9.82 0 top
U1  69.52,18.71 0 top
U2  26.97,13 180 top
U3  38.4,13 180 top
VD1  24.43,28.88 90 top
VD2  30.78,28.88 90 top
VD3  37.13,28.88 90 top
VD4  61.26,28.88 90 top
VD5  67.61,28.88 90 top
VD6  73.96,28.88 90 top

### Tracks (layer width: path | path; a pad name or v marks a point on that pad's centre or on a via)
3V3
  Top 0.203: R3.1 R5.1 R7.1 65.07,12.37 C7.1
  Bottom 0.203: IC1.OUT 56.81,14.59 57.13,14.27 57.13,11.73 57.77,11.1 61.26,11.1 R7.1
5V_A  (via drill 0.35)
  Top 0.406: v29.51,50.78 OUT1.1
  Bottom 0.406: SJ28.1 29.32,50.97 v29.51,50.78
  pour Top: 13,42.21 13,62.53 86.66,62.53 87.93,61.26 87.93,42.21
5V_B  (via drill 0.35)
  Top 0.406: v29.51,73.96 OUT10.1
  Bottom 0.406: SJ29.1 29.32,73.83 29.51,73.64 v29.51,73.96 | OUT10.1 24.43,78.09 LED3.A
  pour Top: 13,85.39 87.93,85.39 87.93,63.8 13,63.8
+5V  (via drill 0.35)
  Top 0.305: v25.7,36.5 25.68,36.52 23.82,36.52
  Top 0.406: R17.2 42.21,21.75 45.07,18.89 Q7.S 45.07,10.46 | 45.07,10.46 45.07,7.6 SV1.4 | v33.32,12.82 33.32,10.46 32.05,9.19 32.05,6.01 SV2.4 | v17.45,29.19 18.08,30.14 19.21,31.27 19.53,31.27 22.03,33.77 22.03,36 22.55,36.52 23.82,36.52 | J10.1 52.37,13 | 52.37,13 R16.1 47.29,10.46 45.07,10.46 | 52.37,13 52.37,13.32 IC1.IN | K1.2 53.01,33.95 v53.01,27.29 | v61.9,38.72 61.9,34.36 58.62,31.08 58.62,30.48 58.72,30.38 R1.1 59.53,26.79 59.53,26.15 59.98,25.69 59.98,24.44 59.99,24.43 v59.99,24.33 | C1.1 65.7,16.68 U1.8 | v19.67,20.94 v15.22,20.94
  Bottom 0.203: SJ9.2 30.18,36.31 30.29,36.42 31.27,36.42 31.38,36.31 SJ11.2 35.89,36.31 36,36.42 36.99,36.42 37.1,36.31 SJ13.2 | R2.1 32.67,22.52 33.94,23.79 40.02,23.79 41.29,22.52 R17.2
  Bottom 0.305: v25.7,36.5 27.42,36.5 SJ9.2
  Bottom 0.406: Q7.S 43.3,12.82 v33.32,12.82 19.48,12.82 18.77,13.54 18.77,13.58 J1.2 17.45,15.54 19.67,17.76 19.67,18.13 18.88,18.92 18.88,19.78 19.5,20.4 19.67,20.4 v19.67,20.94 | v53.01,27.29 54.96,27.29 55.06,27.19 58.31,27.19 R1.1 | SJ20.2 62.03,38.85 v61.9,38.72 | v59.99,24.33 60.87,24.33 61.38,23.82 64.41,23.82 U1.8 | LED2.A 85.39,27.11 82.05,23.77 67.77,23.77 66.52,22.52 U1.8 | U1.8 63.8,20.62 60.48,20.62 59.87,21.23 55.75,21.23 55.14,20.62 55.12,20.64 53.12,20.64 52.52,21.25 47.15,21.25 46.54,20.64 45.5,20.64 44.89,21.25 44.75,21.25 44.11,20.62 R17.2 | v17.45,29.19 17.45,28.88 K2.2 14.9,26.34 14.9,21.25 v15.22,20.94
  pour Top: 13,39.67 87.93,39.67 87.93,2.84 13,2.84
+15V  (via drill 0.35)
  Top 0.305: v73.96,36.81 73.64,36.5 68.25,36.5 67.61,35.86 v67.61,33.5
  Top 0.356: v26.18,33.5 29.17,36.5 43.16,36.5 v43.48,36.18 | v46.02,36.5 47.92,36.5 48.56,37.13
  Top 0.508: 48.56,37.13 v52.37,37.13
  Bottom 0.203: SJ7.2 v73.96,36.81
  Bottom 0.356: 58.51,37.13 59.15,36.5 60.52,36.5 61.26,35.75 61.26,34.89 62.39,33.76 62.91,33.76 SJ14.2 63.78,33.5 64.23,33.95 67.18,33.95 67.61,33.53 v67.61,33.5 SJ16.2 | 42.84,33.95 41.68,33.95 41.23,33.5 SJ12.2 37.47,33.5 37.02,33.95 35.97,33.95 35.52,33.5 SJ10.2 33.05,33.5 32.98,33.43 31.83,33.43 31.31,33.95 30.25,33.95 29.8,33.5 SJ8.2 v26.18,33.5 25.72,33.5 25.27,33.95 23.27,33.95 19.84,30.53 19.51,30.53 18.91,29.93 18.91,28.75 18.08,27.92 | 22.5,30.01 23.9,31.41 24.96,31.41 25.7,32.16 25.7,33.03 25.85,33.17 | 42.84,33.95 42.84,34.06 43.48,34.7 v43.48,36.18 | 48.56,35.86 48.56,34.7 47.82,33.95 42.84,33.95
  Bottom 0.406: SJ26.1 16.18,22.84 16.49,22.52 18.08,22.52 | 21.26,28.24 21.52,28.24 22.5,29.22 22.5,30.01 | 25.85,33.17 v26.18,33.5 | SJ50.1 54.09,37.31 54.27,37.13
  Bottom 0.508: 58.51,37.13 54.27,37.13 v52.37,37.13 49.83,37.13 48.56,35.86
  Bottom 0.813: J1.3 14.9,16.18 18.08,19.35 18.08,22.52 18.08,27.92 18.4,28.24 21.26,28.24 | v43.48,36.18 45.7,36.18 v46.02,36.5
B1  (via drill 0.35)
  Top 0.203: v55.55,19.98 55.55,26.85 54.54,27.85 v54.54,29.19 55.23,29.88 55.23,33 56.18,33.95 K1.9
  Bottom 0.203: v54.54,29.19 55.24,29.89 57.05,29.89 57.31,30.14 VD4.A 63.98,30.14 SJ5.2 | R8.1 R7.2 66.32,9.82 63.8,12.35 63.8,16.83 63.06,17.57 60.84,17.57 59.57,18.84 58.88,18.84 57.74,19.98 v55.55,19.98 53.02,19.98 52.56,20.44 47.74,20.44 47.28,19.98 SV1.5 41.29,19.98 40.14,18.84 39.16,18.84 U3.3
B2  (via drill 0.35)
  Top 0.203: v25.7,24.33 25.7,24.19 24.56,23.05 24.56,22 25.43,21.13 26.17,21.13 26.84,20.46 26.84,19.51 25.7,18.37 U2.3
  Bottom 0.203: SJ2.2 25.06,30.78 VD1.A 23.16,28.88 23.16,26.97 | K2.9 23.16,26.97 | 23.16,26.97 23.38,26.97 23.94,26.41 24.99,26.41 25.7,25.7 v25.7,24.33 | SV2.5 30.77,19.97 29.84,19.97 28.71,18.84 27.73,18.84 U2.3
DAC_L
  Bottom 0.203: MOD1.5 57.49,14.23 57.49,14.62 56.56,15.54 52.05,15.54 51.1,16.49 J13.3
DAC_R
  Bottom 0.203: MOD1.4 58.72,15.54 58.09,15.54 56.18,17.45 J13.1
DIN
  Top 0.203: SV1.3 39.67,6.65 U3.6
  Bottom 0.203: J10.2 51.1,4.75 43.83,4.75 42.68,5.89 41.74,5.89 40.59,4.75 SV1.3
DOUT
  Bottom 0.203: SJ1.2 23.98,9.19 U2.5 | SJ1.2 26.52,5.56 SV2.2 | SJ1.2 26.52,7.47 26.97,7.92 28.24,7.92 28.88,7.29 42.84,7.29 44.11,6.01 J10.4
G1  (via drill 0.35)
  Top 0.203: R6.1 70.15,8.55 70.15,13.63 69.52,14.27 69.52,22.84 68.71,23.64 68.05,23.64 67.1,24.59 67.1,25.54 67.97,26.4 68.11,26.4 68.81,27.11 68.81,28.1 67.61,29.31 VD5.A | U3.1 v42.21,11.41
  Bottom 0.203: SJ6.2 68.25,30.78 VD5.A | R6.1 R5.2 66.34,8.55 57.77,8.55 56.5,9.82 56.5,13 55.86,13.63 52.36,13.63 50.14,11.41 v42.21,11.41 | SV1.8 36.01,18.56 36.01,16.35 36.67,15.69 41.09,15.69 U3.1
G2  (via drill 0.35)
  Top 0.203: v26.97,21.25 26.97,21.87 27.1,22 27.1,23.58 28.55,25.03 28.55,27.08 30.78,29.31 VD2.A
  Bottom 0.203: SJ3.2 33.5,30.14 VD2.A | v26.97,21.25 24.43,21.25 SV2.8 24.43,18.71 24.43,16.18 25.06,15.54 29.51,15.54 U2.1
GND
  Top 0.406: C13.2 23.03,21.87 24.41,20.5 24.41,18.05 U2.4 23.16,10.91 24.38,9.7 24.38,8.68 23.16,7.47 SV2.1 | C12.2 34.46,21.62 33.34,20.5 33.34,18.08 34.59,16.84 U3.4 34.59,10.91 33.37,9.7 33.37,8.68 34.59,7.47 SV1.1 | J7.3 72.06,38.4 76.5,38.4 J8.3 78.9,36 78.9,33.77 81.26,31.41 81.26,29.19 82.85,27.61 C6.2 C5.2 C4.2 82.85,13 81.72,11.87 81.4,11.87 78.9,9.37 78.9,9.05 MOD1.10 | R18.2 44.75,32.69 47.92,29.51 Q9.3 51.1,25.07 51.1,23.16 52.37,21.89 C2.2 J13.2 54.91,16.49 IC1.GND | C1.2 C3.2
  Bottom 0.203: SJ27.2 21.7,23.34
  Bottom 0.406: J3.3 J4.3 J5.3 R18.2 | C13.2 22.52,22.52 21.7,23.34 | J1.1 23.16,14.9 | 23.16,14.9 34.59,14.9 | 34.59,14.9 42.84,14.9 47.92,19.98 52.37,19.98 53.01,19.35 53.64,19.35 | J6.3 67.61,37.77 68.1,37.28 69.66,37.28 70.15,37.77 J7.3 | J10.3 49.83,10.46 51.1,11.73 54.91,11.73 | 54.91,11.73 54.91,9.19 56.81,7.29 MOD1.7 | IC1.GND 54.91,11.73 | C4.2 81.58,16.18 73.33,16.18 | C3.2 72.18,19.22 73.33,18.08 73.33,16.18 | 73.33,16.18 U1.4 | C1.2 59.97,16.3 59.87,16.2 58.84,16.2 58.11,16.93 58.11,18.69 57.45,19.35 55.95,19.35 55.85,19.25 55.24,19.25 55.14,19.35 53.64,19.35 | J13.2 53.64,19.35 | 73.33,16.18 70.33,16.18 69.57,15.41 69.57,13.56 C7.2 | U3.4 34.59,14.9 | U2.4 23.16,14.9 | SJ51.2 47.92,29.7 Q9.3
  pour Bottom: 14.27,2.84 87.93,2.84 87.93,39.67 13,39.67 13,2.84
GND_A
  pour Bottom: 13,40.94 87.93,40.94 87.93,62.53 13,62.53
GND_B
  pour Bottom: 13,63.8 87.93,63.8 87.93,85.39 13,85.39
N$4
  Top 0.203: SV1.2 37.13,6.65 U3.5 | SV2.3 28.24,6.65 U2.6
  Bottom 0.203: SV1.2 35.23,6.65 SJ1.1 28.24,5.83 SV2.3
N$5
  Top 0.406: LED3.K 23.06,79.12 24.73,80.79 24.73,82.47 23.62,83.59 23.34,83.59 23.06,83.87 R20.1
N$6
  Bottom 0.203: R9.1 LED2.K
N$7
  Top 0.203: R4.2 75.55,6.33 75.55,11.1 76.82,12.37 MOD1.12 79.67,14.9 C4.1
N$8
  Top 0.203: R6.2 75.19,8.52 75.19,13.28 76.82,14.9 MOD1.13 80.31,18.08 C5.1
N$9
  Bottom 0.406: C2.1 58.09,24.43 R1.2 58.72,23.16 MOD1.1 62.02,22.52 C3.1
N$10
  Bottom 0.203: R13.2 Q4.G 61.9,26.97 VD4.C
N$11
  Top 0.406: OUT1.4 32.28,57.88 37.59,52.57 37.59,46.71 36.47,45.59 35.91,45.59 OUT2.2
  Bottom 0.406: SJ30.2 38.42,48.66 38.42,47.54 36.47,45.59 35.91,45.59 OUT2.2
N$12
  Top 0.406: OUT2.4 35.07,43.63 36.47,43.63 40.38,47.54 40.38,56.76 41.5,57.88 42.06,57.88 OUT3.2
  Bottom 0.406: SJ31.2 39.82,54.81 39.82,56.2 41.5,57.88 42.06,57.88 OUT3.2
N$14  (via drill 0.35)
  Top 0.406: J5.1 43.48,31.41 v43.48,26.66
  Bottom 0.203: SJ49.2 43.66,25.7
  Bottom 0.406: 43.66,25.7 Q9.2 | v43.48,26.66 SJ49.2
N$16
  Top 0.406: LED4.K 23.06,53.69 23.06,53.97 24.73,55.65 24.73,59.28 23.62,60.4 23.34,60.4 23.06,60.68 R21.1
N$17
  Bottom 0.203: R15.2 Q6.G 74.59,26.97 VD6.C
N$18
  Top 0.406: R18.1 44.75,25.7 Q8.2
  Bottom 0.203: Q3.D 41.58,30.59 SJ4.1
  Bottom 0.406: Q3.D 43.48,28.88 R18.1 | SJ49.1 43.59,24.5 44.06,24.5 44.13,24.43 Q8.2 47.29,23.16 Q9.1
N$19
  Bottom 0.203: Q8.1 43.87,24.04 42.74,24.04 41.72,25.07 R12.2 40.3,25.7 Q3.G 39.67,27.61 VD3.C
N$21  (via drill 0.35)
  Top 0.203: v55.86,32.05 56.81,32.05 J2.2
  Bottom 0.203: SJ21.2 55.86,30.91 v55.86,32.05 | SJ24.1 51.88,33.32 52.77,34.21 57.39,34.21 58.4,35.22 J2.2
N$22
  Bottom 0.203: J4.1 36.5,32.23 SJ3.1 35.04,29.06 Q2.D
N$23
  Bottom 0.203: R11.2 33.95,25.7 Q2.G 33.32,27.61 VD2.C
N$24
  Top 0.203: R14.1 69.52,26.34 Q5.S 69.52,33.95 70.78,35.22 J7.2
  Bottom 0.356: SJ16.1 SJ17.1 71.23,35.41 J7.2
N$25  (via drill 0.35)
  Top 0.203: J8.2 75.87,33.95 Q6.S 75.87,26.34 R15.1 74.59,19.98 v72.49,17.88
  Bottom 0.203: SJ19.1 70.82,38.85 70.93,38.96 71.91,38.96 72.02,38.85 SJ7.1 74.46,38.85 75.55,37.77 75.55,36.18 76.5,35.22 J8.2 | v72.49,17.88 71.67,17.88 SJ46.2
N$26
  Bottom 0.203: J3.1 30.59,32.69 SJ2.1 28.69,29.06 Q1.D
N$27
  Top 0.203: Q1.G 27.61,25.7 R10.2
  Bottom 0.203: Q1.G 26.97,27.61 VD1.C
N$29
  Bottom 0.203: SJ25.2 55.18,32.77 55.18,31.79 54.17,30.78 SJ22.1
  Bottom 0.406: K1.6 53.64,28.24 | 53.64,28.24 K1.5 | SJ22.1 54.09,29.96 53.64,29.51 53.64,28.24
N$32
  Bottom 0.203: R14.2 Q5.G 68.25,26.97 VD5.C
N$34  (via drill 0.35)
  Top 0.406: K1.10 54.91,38.4 53.64,37.13 53.64,35.86 v53.01,35.22
  Bottom 0.406: SJ51.1 J9.3 48.88,32.69 49.61,33.42 50.55,33.42 | 50.55,33.42 SJ24.2 | v53.01,35.22 52.37,34.59 51.1,34.59 50.55,34.04 50.55,33.42
N$35
  Bottom 0.406: J9.1 47.92,38.4 K1.1 SJ50.2
N$36  (via drill 0.35)
  Top 0.406: J9.2 50.47,32.05 v51.1,32.05
  Bottom 0.406: SJ22.2 52.37,30.78 52.37,32.05 | 52.37,32.05 52.37,33.16 52.52,33.32 SJ23.2 | v51.1,32.05 52.37,32.05
N$37
  Top 0.203: R13.1 63.16,26.34 Q4.S 63.16,32.37 65.7,34.91 J6.2
  Bottom 0.356: SJ14.1 SJ15.1 65.52,35.41 J6.2
N$41  (via drill 0.35)
  Top 0.203: R11.1 32.69,26.97 Q2.S v32.69,34.14
  Bottom 0.203: v32.69,34.14 33.69,34.14 SJ10.1 SJ11.1 34.14,35.22 J4.2
N$42
  Top 0.203: R10.1 26.34,26.97 Q1.S 26.34,30.78 J3.2
  Bottom 0.203: SJ8.1 SJ9.1 30.59,35.41 J3.2
N$43
  Top 0.406: J11.2 24.43,34.52 23.12,33.21 23.12,24.56 21.66,23.09 21.66,20.39 K2.6 K2.5
N$44  (via drill 0.35)
  Top 0.203: Q7.D 47.61,20.94 v49.83,23.16 | v64.44,28.88 64.44,33.14 65.33,34.03 66.2,34.03 66.9,34.73 66.9,35.78 66.97,35.86 66.97,36.03 v66.68,36.33
  Bottom 0.203: SJ17.2 66.66,36.31 | 66.66,36.31 66.31,36.31 66.2,36.42 65.21,36.42 65.1,36.31 SJ15.2 SJ20.1 64.2,37.95 65.21,38.96 67.06,38.96 68.07,37.95 SJ19.2 | v49.83,23.16 52.37,25.7 57.74,25.7 58.25,26.21 59.23,26.21 60.07,27.05 60.07,28.1 60.77,28.8 61.91,28.8 62.77,27.93 63.56,27.93 64.11,28.48 64.11,28.55 v64.44,28.88 | v66.68,36.33 66.66,36.31
N$45  (via drill 0.35)
  Top 0.406: v22.21,25.07 22.21,26.39 22.36,26.54 22.36,28.41 21.26,29.51 K2.10
  Bottom 0.406: SJ27.1 22.21,25.2 v22.21,25.07 | K2.10 23.8,32.69 J11.3
N$46  (via drill 0.35)
  Top 0.406: v16.49,25.38 16.49,25.75 17.28,26.54 17.28,27.77 K2.1
  Bottom 0.406: SJ26.2 16.18,25.07 v16.49,25.38 | J11.1 22.03,35.36 22.03,33.74 19.35,31.06 18.28,31.06 16.73,29.51 K2.1
N$47
  Top 0.406: OUT3.4 44.85,57.88 50.44,52.29 50.44,46.71 49.32,45.59 48.76,45.59 OUT4.2
  Bottom 0.406: SJ32.2 51.28,48.66 51.28,47.54 49.32,45.59 48.76,45.59 OUT4.2
N$48
  Top 0.406: INP.2 16.07,45.59 14.4,47.27 14.4,48.38 18.03,52.01 23.62,52.01 27.81,56.2 27.81,56.76 28.93,57.88 29.48,57.88 OUT1.2
N$49
  Top 0.406: OUT10.4 32.28,80.51 37.59,75.2 37.59,69.06 36.47,67.94 35.91,67.94 OUT11.2
  Bottom 0.406: SJ38.2 38.42,71.01 38.42,70.17 35.91,67.66 OUT11.2
N$50
  Top 0.406: OUT4.4 46.25,45.31 47.92,43.63 49.04,43.63 53.23,47.82 53.23,56.76 54.35,57.88 54.91,57.88 OUT5.2
  Bottom 0.406: SJ33.2 52.4,54.81 52.4,55.93 54.35,57.88 54.91,57.88 OUT5.2
N$51
  Top 0.406: OUT5.4 57.7,57.88 63.01,52.57 63.01,46.71 61.9,45.59 61.34,45.59 OUT6.2
  Bottom 0.406: SJ34.2 63.85,48.66 63.85,47.54 61.9,45.59 61.34,45.59 OUT6.2
N$54
  Top 0.406: OUT11.4 33.4,67.66 34.79,66.26 36.47,66.26 40.38,70.17 40.38,79.4 41.5,80.51 42.06,80.51 OUT12.2
  Bottom 0.406: SJ39.2 39.82,77.72 39.82,78.56 40.94,79.67 41.22,79.67 42.06,80.51 OUT12.2
N$55
  Top 0.406: OUT7.4 70.28,57.88 75.87,52.29 75.87,46.43 74.75,45.31 74.19,45.31 OUT8.2
  Bottom 0.406: SJ36.2 76.7,48.66 76.7,47.82 74.19,45.31 OUT8.2
N$56
  Bottom 0.406: 63.85,50.9 63.85,52.01 64.83,52.99 | 63.85,50.9 63.85,49.78 SJ34.1 | 64.83,52.99 64.97,53.13 64.97,53.69 SJ35.1 | 76.84,52.43 77.54,53.13 77.54,53.69 SJ37.1 | 76.84,52.43 76.7,52.29 76.7,49.78 SJ36.1 | 64.83,52.99 65.25,52.57 76.42,52.57 | 76.42,52.57 76.7,52.57 76.84,52.43 | 76.42,52.57 76.42,56.48 79.78,59.84 80.89,59.84 82.57,58.16 82.85,58.16 OUT9.4 | 38.42,52.01 38.42,49.78 SJ30.1 | 39.4,52.99 39.54,53.13 39.54,53.69 SJ31.1 | 39.4,52.99 38.42,52.01 | 39.4,52.99 39.82,52.57 43.17,52.57 46.25,49.5 51,49.5 SJ32.1 51.28,49.5 56.03,49.5 57.42,50.9 | INP.4 20.26,52.01 38.42,52.01 | 57.42,50.9 63.85,50.9 | SJ33.1 52.55,53.64 56.18,53.64 57.45,52.37 57.42,52.34 57.42,50.9
N$57
  Top 0.406: OUT8.4 71.67,45.31 73.35,43.63 74.47,43.63 78.38,47.54 78.38,56.48 80.06,58.16 OUT9.2
  Bottom 0.406: SJ37.2 77.82,54.81 77.82,55.93 80.06,58.16 OUT9.2
N$58
  Top 0.406: OUT12.4 44.85,80.51 46.53,78.84 46.53,74.09 43.73,71.29 43.73,67.94 45.41,66.26 47.09,66.26 48.48,67.66 OUT13.2
  Bottom 0.406: SJ40.2 51.28,71.01 51.28,69.34 49.88,67.94 48.76,67.94 OUT13.2
N$59
  Top 0.406: INP1.2 16.07,68.5 14.4,70.17 14.4,71.29 17.75,74.65 23.34,74.65 27.81,79.12 27.81,79.4 28.93,80.51 29.48,80.51 OUT10.2
N$60
  Top 0.406: OUT13.4 45.97,67.94 44.29,69.62 44.29,71.01 53.79,80.51 54.91,80.51 OUT14.2
  Bottom 0.406: SJ41.2 52.4,76.6 52.95,76.6 53.51,77.16 53.51,78 52.67,78.84 52.67,79.12 54.07,80.51 54.91,80.51 OUT14.2
N$61
  Top 0.406: OUT6.4 58.82,45.31 60.5,43.63 61.9,43.63 65.81,47.54 65.81,56.76 66.92,57.88 67.48,57.88 OUT7.2
  Bottom 0.406: SJ35.2 65.25,54.81 65.25,56.2 66.92,57.88 67.48,57.88 OUT7.2
N$62
  Top 0.406: OUT14.4 57.7,80.51 63.01,75.2 63.01,69.34 61.34,67.66 OUT15.2
  Bottom 0.406: SJ42.2 63.85,71.01 63.85,70.17 61.34,67.66 OUT15.2
N$65
  Bottom 0.406: OUT17.2 74.19,67.94 75.31,67.94 76.7,69.34 76.7,71.01 SJ44.2 76.42,71.29 75.87,71.29 75.03,72.13 75.03,75.76 70.28,80.51 OUT16.4
N$66  (via drill 0.35)
  Top 0.406: v56.18,72.69 56.18,75.23 55.55,75.87 51.1,75.87 v51.1,76.44
  Bottom 0.406: 64.27,77.86 64.41,78 64.69,77.72 64.69,77.44 64.97,77.44 SJ43.1 | 64.27,77.86 63.57,77.16 63.57,76.04 63.85,75.76 63.85,72.41 SJ42.1 | 76.84,76.18 77.54,76.88 SJ45.1 | 76.84,76.18 76.7,76.04 76.7,72.41 SJ44.1 | 76.84,76.18 76.42,76.6 76.42,79.12 76.56,79.26 | 76.56,79.26 79.5,82.19 81.17,82.19 82.85,80.51 OUT18.4 | 64.27,77.86 63.85,78.28 63.85,79.12 63.99,79.26 | 63.99,79.26 66.92,82.19 73.63,82.19 76.56,79.26 | 38.42,74.92 38.42,72.41 SJ38.1 | 39.4,75.9 39.54,76.04 39.54,76.6 SJ39.1 | 39.4,75.9 38.42,74.92 | 51,77.72 46.81,77.72 44.57,75.48 39.82,75.48 39.4,75.9 | 51,77.72 51.1,77.72 | 51.1,77.72 52.12,77.72 SJ41.1 | 38.42,74.92 20.26,74.92 16.35,71.01 INP1.4 | 51,77.72 51,79.12 54.07,82.19 58.26,82.19 61.06,79.4 63.85,79.4 63.99,79.26 | SJ40.1 55.99,72.19 56.18,72.37 v56.18,72.69 | v51.1,76.44 51.1,77.72
N$67
  Top 0.406: OUT17.4 71.4,67.94 69.72,69.62 69.72,71.01 79.22,80.51 80.06,80.51 OUT18.2
  Bottom 0.406: SJ45.2 77.82,77.72 77.82,78.84 79.5,80.51 80.06,80.51 OUT18.2
N$68
  Bottom 0.406: 65.95,76.74 66.37,77.16 66.37,78.28 65.81,78.84 65.81,79.12 66.37,79.67 66.65,79.67 67.48,80.51 OUT16.2 | 65.95,76.74 65.81,76.6 65.25,76.6 SJ43.2 | 65.95,76.74 66.37,76.32 66.37,70.73 61.9,66.26 60.22,66.26 58.82,67.66 OUT15.4
N$69
  Top 0.406: 24.73,45.59 18.87,45.59 INP.1 | 24.73,45.59 26.13,46.98 26.13,47.82 C8.1 | 24.73,45.59 26.41,43.91 26.41,43.07 C9.1
  Bottom 0.406: SJ28.2 C8.1
N$70
  Bottom 0.203: U1.1 65.25,15.36 SJ47.2
N$73
  Top 0.406: 24.87,68.64 26.13,69.9 26.13,70.73 C10.1 | 24.87,68.64 24.73,68.5 18.87,68.5 INP1.1 | C11.1 26.13,65.7 25.01,66.82 25.01,68.5 24.87,68.64
  Bottom 0.406: SJ29.2 C10.1
N$74  (via drill 0.35)
  Top 0.203: R9.2 79.99,28.79 81.45,27.33 81.45,18.21 v81.58,18.08 | v66.97,19.98 v66.97,18.49
  Bottom 0.203: SJ48.2 SJ47.1 66.97,18.27 v66.97,18.49 | v81.58,18.08 78.12,18.08 77.61,18.59 73.46,18.59 72.07,19.98 v66.97,19.98
PB0
  Bottom 0.152: U1.5 73.35,22.5 75.48,22.5 76.7,21.28 78.84,21.28 80.82,23.26 82.65,23.26 86.61,27.22 86.61,27.99 85.85,28.75 78.53,28.75 Q6.D
  Bottom 0.203: Q6.D 78.41,29.32 SJ18.1 76.95,32.5 J8.1
PB1
  Top 0.203: U1.6 72.06,23.79 Q5.D 72.06,32.05 J7.1
  Bottom 0.203: SJ6.1 71.23,32.5 J7.1 J12.1
PB2
  Top 0.203: U1.7 65.7,25.07 Q4.D
  Bottom 0.203: J12.2 73.33,33.95 70.78,33.95 69.52,32.69 J6.1 65.52,32.5 SJ5.1 65.52,29.06 Q4.D
PB3  (via drill 0.35)
  Top 0.203: U1.2 66.97,13.63 65.05,13.63 63.15,11.73 v62.53,11.73
  Bottom 0.203: U1.2 68.69,15.36 SJ48.1 SJ46.1 | Q7.G 47.61,12.68 49.83,14.9 R16.2 49.83,18.71 50.47,19.35 51.73,19.35 52.37,18.71 52.37,16.18 52.65,15.9 56.71,15.9 59.1,13.51 59.83,13.51 60.5,12.84 60.5,11.86 60.62,11.73 v62.53,11.73
PB4
  Top 0.203: C6.1 77.64,23.67 76.66,23.67 74.95,21.96 74.95,13.99 73.96,13 R8.2
  Bottom 0.203: U1.3 70.78,13 R8.2
PWR1
  Top 0.203: R17.1 41.07,21.13 41.07,18.59 41.73,17.93 42.67,17.93 43.33,17.27 43.33,10.31 U3.8
  Bottom 0.203: R17.1 C12.1
PWR2  (via drill 0.35)
  Top 0.203: v32.05,18.08 32.05,10.46 U2.8
  Bottom 0.203: C13.1 R2.2 29.64,21.13 31.25,21.13 32.05,20.33 v32.05,18.08
Q8_POWER
  Top 0.203: R12.1 39.03,26.97 Q3.S
  Top 0.406: J5.2 39.03,32.05 Q3.S
  Bottom 0.203: J5.2 39.86,35.22 SJ13.1
  Bottom 0.406: SJ12.1 SJ13.1 | Q8.3 45.08,27.91 42.09,27.91 42.01,27.83 41.14,27.83 40.09,28.88 Q3.S
R1  (via drill 0.35)
  Top 0.203: v40.94,10.46 40.94,15.54 U3.2 SV1.6 | R4.1 71.9,7.77 71.9,15.37 71.86,15.41 71.86,18.14 72.21,18.49 72.21,22.99 72.76,23.54 72.76,28.1 73.96,29.31 VD6.A
  Bottom 0.203: SJ18.2 75.23,30.78 74.59,30.14 VD6.A | R4.1 R3.2 66.34,6.01 54.91,6.01 53.64,7.29 44.43,7.29 43.8,7.92 41.58,7.92 40.94,8.55 v40.94,10.46
R2
  Top 0.203: 29.51,18.08 30.78,18.08 32.05,19.35 32.05,21.89 33.19,23.03 33.19,23.05 33.94,23.79 33.95,23.79 34.59,24.43 34.59,26.27 34.9,26.58 34.9,27.21 36.17,28.48 36.17,29.18 VD3.A | 29.51,18.08 28.24,19.35 SV2.6 | U2.2 29.51,18.08
  Bottom 0.203: SJ4.2 39.86,30.14 VD3.A
SPK1  (via drill 0.35)
  Top 0.203: MOD1.6 58.09,9.82 57.45,10.46 v57.45,26.34 | v54.27,26.34 54.27,27.61 53.91,27.98 53.91,29.77 53.96,29.82 53.96,32.05 v53.91,32.05 54.19,32.33 54.19,34.37 54.54,34.73 54.54,36.25 55.1,36.81 58.35,36.81 59.31,37.77 J2.1
  Bottom 0.203: v57.45,26.34 v54.27,26.34 | v53.91,32.05 53.91,33.14 SJ23.1
SPK2  (via drill 0.35)
  Top 0.203: MOD1.8 60.62,6.01 60.62,25.7 59.99,26.34 59.99,30.14 v59.35,30.78
  Bottom 0.203: SJ25.1 SJ21.1 v59.35,30.78

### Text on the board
Top: Top | Top | Top
Bottom: Bottom | Bottom | Bottom | Bottom
Dimension: ~ | v-cut | v-cut | ~ | v-cut | v-cut | If v-cut is not possible, then / it should be made as a part | If v-cut is not possible, then / it should be made as a part
tPlace: Out 1 | Out 3 | Out 5 | Out 7 | Out 9 | Inp | Kai & Hardi | 10.11.18 | Out 2 | Out 4 | Out 6 | Out 8 | Out 1 | Out 3 | Out 5 | Out 7 | Out 9 | Inp | Kai & Hardi | 10.11.18 | Out 2 | Out 4 | Out 6 | Out 8 | + | V 1.0 | 10.11.18 | 5V | S3PO-Modul | Kai & Hardi | GND | 8V-16V
bPlace: Kai & Hardi / 10.11.18 | Kai & Hardi / 10.11.18 | 5V | Sound, Signal, Servo and Power / Output Modul with WS2811 | GND | 8V-16V | Kai & Hardi / 10.11.18

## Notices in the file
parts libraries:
SparkFun-Capacitors: Licensing: Creative Commons ShareAlike 4.0 International - https://creativecommons.org/licenses/by-sa/4.0
